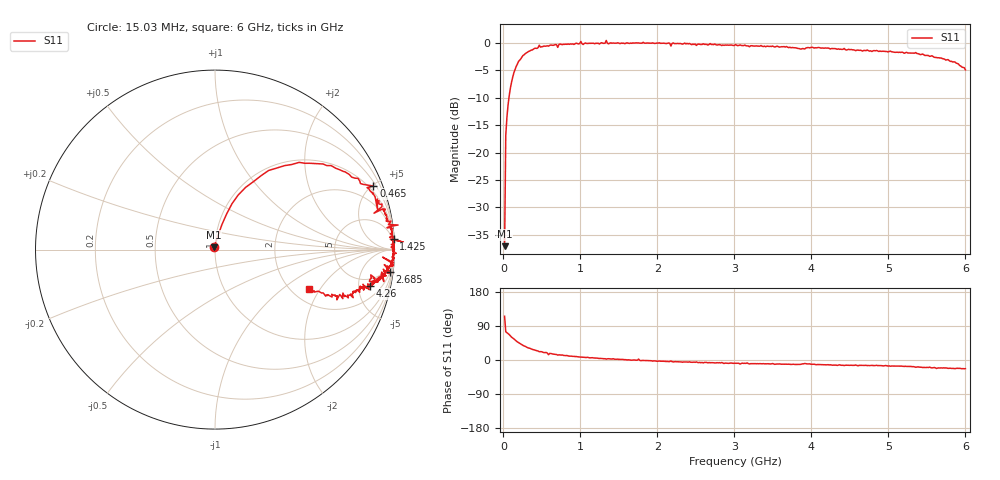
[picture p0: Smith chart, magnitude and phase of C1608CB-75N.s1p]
!	Network	Analyzer	HP8753E.07.74:	Oct	30	2002	Serial	No.	JP38451487
!	Hewlett-Packard
!	28	Aug	2009	8:23:50
!	Frequency	S11
#	HZ	S	RI	R	50
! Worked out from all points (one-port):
!   400 points, 15.03 MHz to 6 GHz, reference 50 ohm
!   lowest |S11| = -37.0 dB at 15.03 MHz (marker M1), VSWR 1.03, Z = 49.4 + j1.25 ohm
!   |S11| at or under -10 dB: start of sweep to 71.69 MHz
!   S11 on the Smith chart (normalised r, x): 15.03 MHz: 0.99, +0.03; 465 MHz: 0.68, +5.09; 1.425 GHz: 2, +34; 2.685 GHz: 2, -16; 4.26 GHz: 3.60, -6.78; 6 GHz: 2.47, -1.60
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1.502992e7  -0.00601 0.0127
3.002985e7  0.038 0.138
6.00297e7  0.0943 0.255
9.002955e7  0.171 0.347
1.95029e8  0.469 0.486
4.650277e8  0.883 0.354
5.550272e8  0.878 0.317
5.850271e8  0.905 0.226
6.150269e8  0.913 0.282
7.650262e8  0.937 0.221
1.005025e9  1.02 0.137
1.035025e9  0.958 0.122
1.245024e9  0.973 0.0678
1.335023e9  1.05 0.0412
1.365023e9  0.977 0.0576
1.425023e9  0.995 0.0583
1.515022e9  0.982 0.0284
2.145019e9  0.994 -0.074
2.175019e9  0.934 -0.0421
2.265019e9  0.985 -0.0795
2.685017e9  0.976 -0.123
3.015015e9  0.954 -0.146
3.765011e9  0.886 -0.175
4.260009e9  0.863 -0.202
4.515007e9  0.845 -0.206
5.265004e9  0.772 -0.237
5.775001e9  0.652 -0.264
6e9  0.524 -0.219
